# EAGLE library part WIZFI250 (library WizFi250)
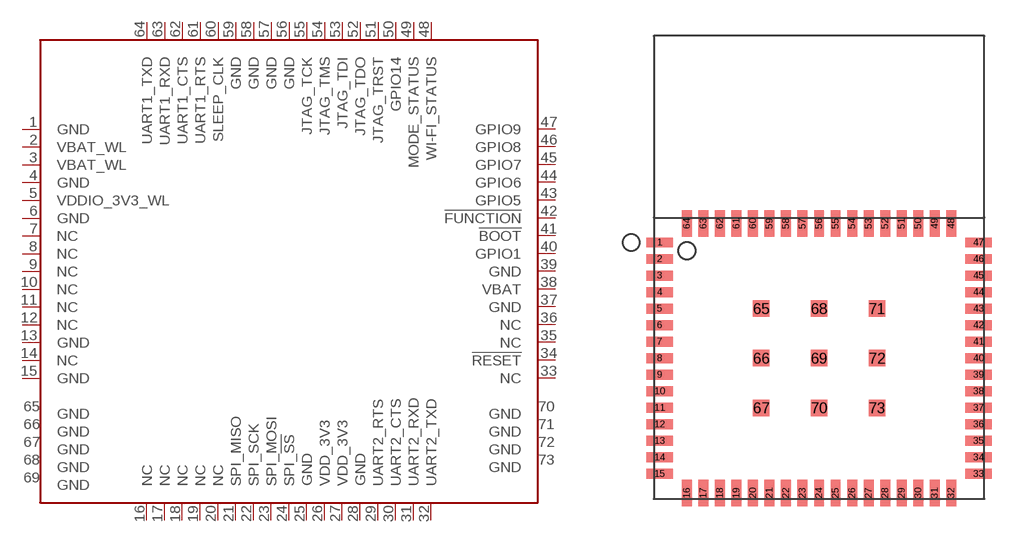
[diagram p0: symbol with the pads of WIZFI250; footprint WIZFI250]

Designator prefix M

## WIZFI250  [WIZFI250]
1  GND  pas
2  VBAT_WL  pas
3  VBAT_WL  pas
4  GND  pas
5  VDDIO_3V3_WL  pas
6  GND  pas
7  NC  pas
8  NC  pas
9  NC  pas
10  NC  pas
11  NC  pas
12  NC  pas
13  GND  pas
14  NC  pas
15  GND  pas
16  NC  pas
17  NC  pas
18  NC  pas
19  NC  pas
20  NC  pas
21  SPI_MISO  pas
22  SPI_SCK  pas
23  SPI_MOSI  pas
24  SPI_!SS  pas
25  GND  pas
26  VDD_3V3  pas
27  VDD_3V3  pas
28  GND  pas
29  UART2_RTS  pas
30  UART2_CTS  pas
31  UART2_RXD  pas
32  UART2_TXD  pas
33  NC  pas
34  !RESET  pas
35  NC  pas
36  NC  pas
37  GND  pas
38  VBAT  pas
39  GND  pas
40  GPIO1  pas
41  !BOOT  pas
42  !FUNCTION  pas
43  GPIO5  pas
44  GPIO6  pas
45  GPIO7  pas
46  GPIO8  pas
47  GPIO9  pas
48  WI-FI_STATUS  pas
49  MODE_STATUS  pas
50  GPIO14  pas
51  JTAG_TRST  pas
52  JTAG_TDO  pas
53  JTAG_TDI  pas
54  JTAG_TMS  pas
55  JTAG_TCK  pas
56  GND  pas
57  GND  pas
58  GND  pas
59  GND  pas
60  SLEEP_CLK  pas
61  UART1_RTS  pas
62  UART1_CTS  pas
63  UART1_RXD  pas
64  UART1_TXD  pas
65  GND  pas
66  GND  pas
67  GND  pas
68  GND  pas
69  GND  pas
70  GND  pas
71  GND  pas
72  GND  pas
73  GND  pas

## Footprint WIZFI250 (pad centres in mm)
smd 1.6 x 0.6: 1 -9.65,1.5; 2 -9.65,0.5; 3 -9.65,-0.5; 4 -9.65,-1.5; 5 -9.65,-2.5; 6 -9.65,-3.5; 7 -9.65,-4.5; 8 -9.65,-5.5; 9 -9.65,-6.5; 10 -9.65,-7.5; 11 -9.65,-8.5; 12 -9.65,-9.5; 13 -9.65,-10.5; 14 -9.65,-11.5; 15 -9.65,-12.5; 33 9.65,-12.5; 34 9.65,-11.5; 35 9.65,-10.5; 36 9.65,-9.5; 37 9.65,-8.5; 38 9.65,-7.5; 39 9.65,-6.5; 40 9.65,-5.5; 41 9.65,-4.5; 42 9.65,-3.5; 43 9.65,-2.5; 44 9.65,-1.5; 45 9.65,-0.5; 46 9.65,0.5; 47 9.65,1.5
smd 0.6 x 1.6: 16 -8,-13.65; 17 -7,-13.65; 18 -6,-13.65; 19 -5,-13.65; 20 -4,-13.65; 21 -3,-13.65; 22 -2,-13.65; 23 -1,-13.65; 24 0,-13.65; 25 1,-13.65; 26 2,-13.65; 27 3,-13.65; 28 4,-13.65; 29 5,-13.65; 30 6,-13.65; 31 7,-13.65; 32 8,-13.65; 48 8,2.65; 49 7,2.65; 50 6,2.65; 51 5,2.65; 52 4,2.65; 53 3,2.65; 54 2,2.65; 55 1,2.65; 56 0,2.65; 57 -1,2.65; 58 -2,2.65; 59 -3,2.65; 60 -4,2.65; 61 -5,2.65; 62 -6,2.65; 63 -7,2.65; 64 -8,2.65
smd 1 x 1: 65 -3.5,-2.5; 66 -3.5,-5.5; 67 -3.5,-8.5; 68 0,-2.5; 69 0,-5.5; 70 0,-8.5; 71 3.5,-2.5; 72 3.5,-5.5; 73 3.5,-8.5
